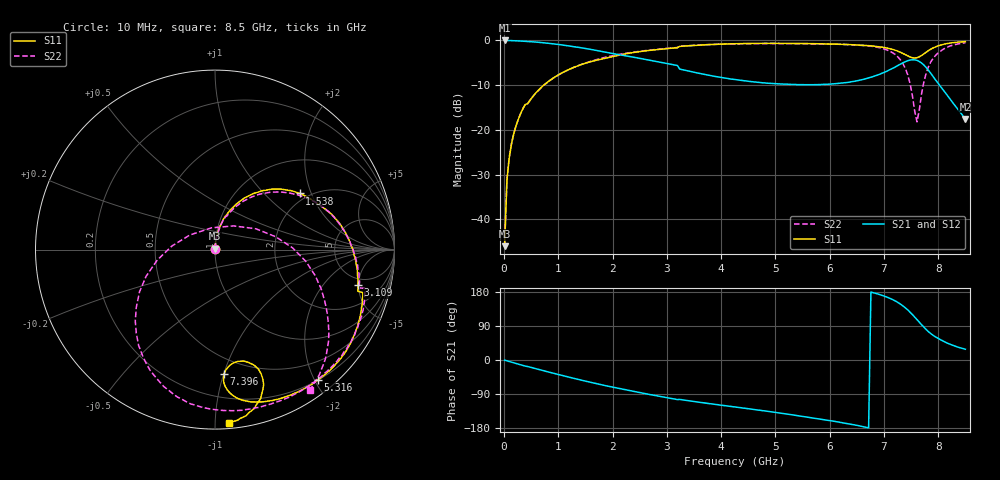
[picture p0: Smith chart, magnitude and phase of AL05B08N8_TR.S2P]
!AVX Corporation
!PN: AL05B08N8*TR
!Description: Air Core Inductor, 8.8nH, 8 Turns
!Agilent Technologies,E5071C,MY46102230,A.09.54
!Date: Mon Sep 03 16:22:29 2012
!Data & Calibration Information:
!Freq	S11:SOLT2(ON)	S21:SOLT2(ON)	S12:SOLT2(ON)	S22:SOLT2(ON)
# Hz S dB R 50
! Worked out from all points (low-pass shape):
!   201 points, 10 MHz to 8.5 GHz, reference 50 ohm
!   highest |S21| = -0.01 dB at 10 MHz (marker M1); lowest = -17.5 dB at 8.5 GHz (marker M2)
!   |S21| within 3 dB of the highest: start of sweep to 2.033 GHz
!   lowest |S11| = -46.0 dB at 10 MHz (marker M3), VSWR 1.01, Z = 50.1 + j0.499 ohm
!   |S11| at or under -10 dB: start of sweep to 730.9 MHz
!   |S22| runs from -45.8 to -0.5 dB; largest |S21 - S12| = 0.011
!   S11 on the Smith chart (normalised r, x): 10 MHz: 1.00, +0.01; 1.538 GHz: 1.80, +1.66; 3.109 GHz: 4.04, -4.89; 5.316 GHz: 0.20, -2.05; 7.396 GHz: 0.38, -1.00; 8.5 GHz: 0.03, -1.08
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1e7  -45.97 82.4  -0.01 -0.4  -0.04 0.1  -45.75 80.0
5.245e7  -31.25 86.4  -0.01 -2.2  0.02 -2.3  -31.15 85.5
9.49e7  -26.23 84.3  -0.03 -4.0  -0.01 -4.1  -26.19 83.7
1.798e8  -20.79 81.1  -0.06 -7.5  -0.04 -7.5  -20.74 80.6
3.0715e8  -16.30 76.1  -0.14 -12.7  -0.12 -12.8  -16.26 75.7
7.741e8  -9.57 60.2  -0.58 -30.0  -0.57 -30.1  -9.60 57.6
1.4533e9  -5.26 36.5  -1.70 -54.2  -1.70 -54.3  -5.24 34.1
1.5382e9  -4.94 33.6  -1.88 -57.1  -1.88 -57.1  -4.89 31.4
2.85415e9  -1.99 -6.8  -4.83 -95.6  -4.83 -95.7  -1.94 -6.4
3.10885e9  -1.73 -14.0  -5.41 -102.3  -5.41 -102.4  -1.66 -12.8
4.255e9  -0.74 -35.2  -8.76 -123.9  -8.76 -123.9  -0.78 -35.2
5.31625e9  -0.67 -51.7  -9.83 -144.9  -9.82 -144.9  -0.72 -59.3
5.6983e9  -0.72 -57.9  -9.89 -153.1  -9.89 -153.1  -0.77 -69.1
6.58975e9  -1.07 -73.7  -8.80 -174.9  -8.80 -174.9  -1.09 -94.3
7.09915e9  -1.82 -83.5  -6.58 163.3  -6.59 163.3  -2.35 -118.4
7.3963e9  -3.19 -85.8  -4.74 137.4  -4.74 137.4  -6.35 -150.8
7.4812e9  -3.71 -83.1  -4.39 126.2  -4.38 126.2  -9.68 -169.5
7.60855e9  -3.86 -75.6  -4.46 106.6  -4.46 106.5  -18.21 99.6
7.7359e9  -2.99 -70.0  -5.51 86.5  -5.51 86.4  -9.21 11.9
7.9057e9  -1.68 -71.1  -8.08 65.1  -8.08 65.1  -4.00 -20.3
8.20285e9  -0.63 -78.5  -12.87 42.3  -12.87 42.2  -1.32 -44.0
8.5e9  -0.27 -85.4  -17.54 28.4  -17.57 28.5  -0.52 -56.0
